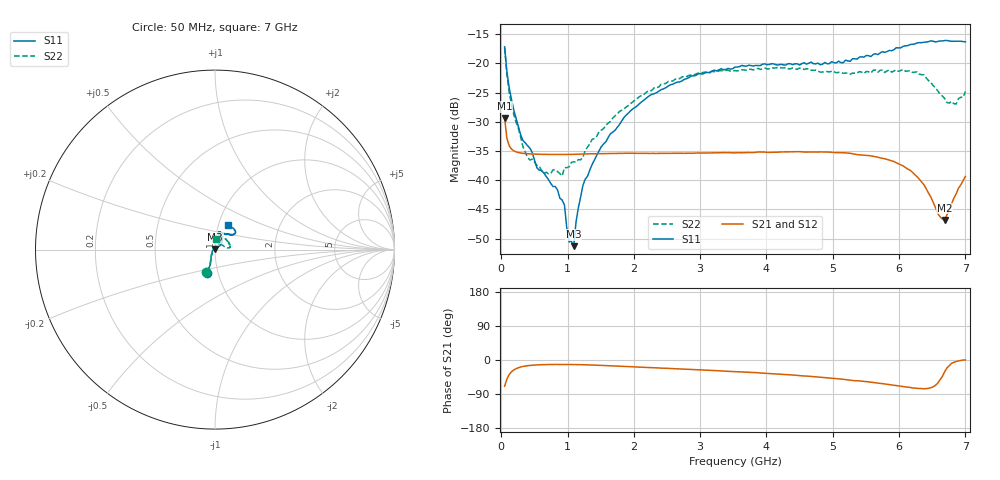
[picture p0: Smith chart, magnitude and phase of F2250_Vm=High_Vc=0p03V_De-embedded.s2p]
! Integrated Device Technology
! Corporate Headquarters
! 6024 Silver Creek Valley Road
! San Jose, CA 95138  USA
! Phone:  1-408-284-8200
! Toll Free:  1-800-223-1366
! Webpage:  http://www.idt.com/
! Timing and RF Division
! 515 Groton Road, Suite 102
! Westford, MA 01886-6024
! Device:  F2250
! Description: Voltage Variable RF Attenuator
! Frequency:  50.0 -  6000.00 MHz
! Package:  3x3 mm Thin QFN Plastic Package: 16 pin
! Ports:  2 RF, 3 DC
!  Pin  1  = GND
!  Pin  2  = NC
!  Pin  3  = RF1  = Port 1
!  Pin  4  = NC
!  Pin  5  = GND
!  Pin  6  = GND
!  Pin  7  = GND
!  Pin  8  = GND
!  Pin  9  = NC
!  Pin 10  = RF2  = Port 2
!  Pin 11  = NC
!  Pin 12  = GND
!  Pin 13  = GND
!  Pin 14  = VCNTRL
!  Pin 15  = VDD
!  Pin 16  = VMODE
! Vcntrl:  0.030 Volts
! Vmode:  +3.300 Volts
! Vdd:  +3.30  Volts
! Current:  1.243 mA
! Data:  The device was measured on a the F2250 evaluation board which has
!  individual transmission lines to the RF pins.  Data was collected
!  using a calibrated network analyzer.  The evaluation board was
!  de-embedded using a TRL calibration technique.
!  The reference plane is the edge of the package pin.
! Misc:  SN 10
!  Action Tracker AT0258
! Date Measured:  2014-11-26
! Date:  2015-10-15  MJV
! Note:
!  Integrated Device Technology supplies this data as a sample of measured
!  data at the package pin for this product.  Your particular data for this
!  product may vary.
!  Data was taken at 25 degrees C.
!  Integrated Device Technology reserves the right to change this data at anytime.
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# GHz S dB R 50
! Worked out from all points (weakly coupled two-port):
!   201 points, 50 MHz to 7 GHz, reference 50 ohm
!   highest |S21| = -29.38 dB at 50 MHz (marker M1); lowest = -46.8 dB at 6.687 GHz (marker M2)
!   lowest |S11| = -51.3 dB at 1.093 GHz (marker M3), VSWR 1.01, Z = 50 + j0.273 ohm
!   |S11| at or under -10 dB: start of sweep to end of sweep
!   |S22| runs from -39.3 to -17.4 dB; largest |S21 - S12| = 6e-05
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0.05  -17.18 -108.5  -29.38 -69.5  -29.38 -69.5  -17.37 -110.6
0.08475  -21.47 -107.4  -32.86 -50.1  -32.86 -50.1  -21.87 -109.0
0.15425  -26.22 -116.6  -34.68 -31.0  -34.68 -31.0  -27.11 -120.7
0.29325  -32.27 -127.5  -35.35 -18.4  -35.35 -18.4  -32.66 -133.4
0.3975  -34.11 -142.2  -35.48 -15.0  -35.48 -15.0  -36.09 -158.4
0.5365  -37.86 -154.7  -35.55 -12.9  -35.55 -12.9  -37.47 -179.9
0.64075  -38.76 -162.5  -35.58 -12.2  -35.58 -12.2  -38.87 160.8
0.91875  -43.41 155.9  -35.60 -11.8  -35.60 -11.8  -39.25 127.9
0.9535  -44.26 171.0  -35.60 -11.8  -35.60 -11.8  -37.83 124.1
1.023  -50.57 140.2  -35.59 -11.9  -35.59 -11.9  -37.71 108.0
1.0925  -51.28 88.8  -35.57 -12.0  -35.57 -12.0  -36.85 98.7
1.12725  -47.13 61.6  -35.56 -12.1  -35.56 -12.1  -36.92 91.7
1.2315  -40.87 40.9  -35.52 -12.5  -35.52 -12.5  -36.07 77.3
1.6485  -32.03 41.3  -35.44 -15.2  -35.44 -15.2  -29.92 60.0
2.37825  -24.75 46.7  -35.40 -21.0  -35.40 -21.1  -24.03 54.0
3.525  -20.65 71.7  -35.32 -30.6  -35.32 -30.6  -21.26 73.0
4.7065  -20.06 72.0  -35.16 -43.9  -35.15 -43.9  -21.21 70.4
5.85325  -17.79 40.5  -36.58 -64.9  -36.58 -64.9  -21.13 23.4
6.27025  -16.53 39.4  -39.39 -74.5  -39.41 -74.6  -21.46 8.6
6.68725  -16.11 47.9  -46.81 -31.0  -46.77 -30.9  -26.02 28.4
6.861  -16.22 54.5  -42.32 -3.7  -42.25 -3.7  -26.96 57.4
7  -16.32 62.4  -39.36 -0.1  -39.32 -0.3  -24.82 83.6
